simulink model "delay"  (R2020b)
settings: Solver=FixedStepAuto  StartTime=0.0  StopTime=10  FixedStep=0.02  RelTol=1e-3
libraries: sldrtlib x1

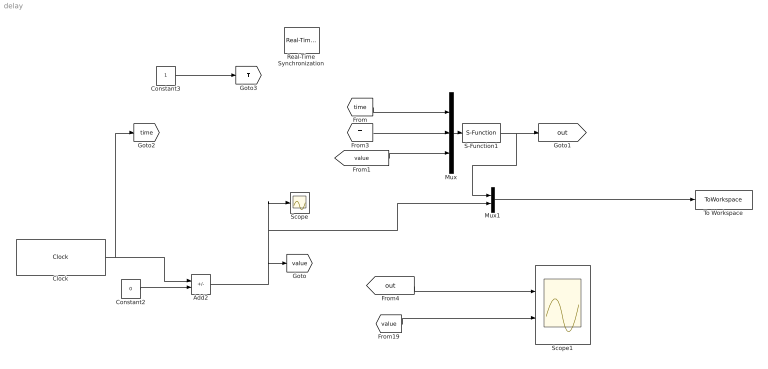
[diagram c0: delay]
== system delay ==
  Add2 : Sum  Inputs=+-
  Clock : Clock
  Constant2 : Constant  Value=0
  Constant3 : Constant
  Mux : Mux  Inputs=3
  Mux1 : Mux  Inputs=2
  Real-Time Synchronization : sldrtlib/Real-Time Synchronization  SampleTime=0.02  MaxMissedTicks=inf  ShowMissedTicks=off  YieldWhenWaiting=off
  S-Function1 : S-Function  FunctionName=modbusComdelay  SFunctionDeploymentMode=off  EnableBusSupport=off
  Scope : Scope
  Scope1 : Scope  NumInputPorts=2
  To Workspace : ToWorkspace  VariableName=simout  SampleTime=-1
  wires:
  Constant2/1 -> Add2/2
  Clock/1 -> [time], Add2/1
  [value] -> Scope1/2
  Add2/1 -> Mux1/2, Scope/1, [value]
  [out] -> Scope1/1
  [value] -> Mux/3
  Mux/1 -> S-Function1/1
  [time] -> Mux/1
  [T] -> Mux/2
  Constant3/1 -> [T]
  S-Function1/1 -> Mux1/1, [out]
  Mux1/1 -> To Workspace/1
